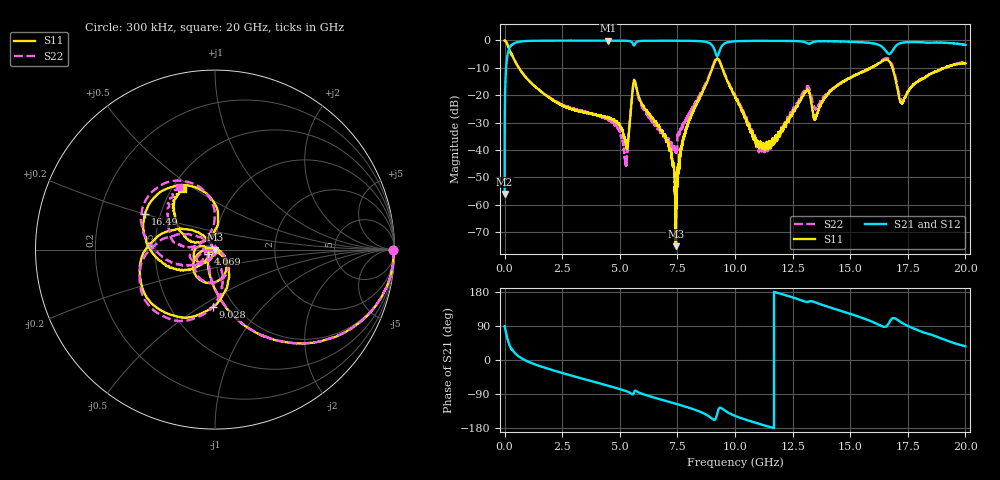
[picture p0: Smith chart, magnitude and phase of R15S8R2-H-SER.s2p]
!{R15S8R2}
!Johanson Technology Inc.
!www.johansontechnology.com
!Test Board Conditions:
!Substrate Type  RO4350B
!Substrate Thickness  20 mil
!Substrate Dk  3.66
!TL Type: GCPW
!TL Trace Width  34 mil
!TL Gap  10 mil
!Electrode orientation  Horizontal
!DUT TOPOLOGY	SERIES
!Mounting Pad LxW  26x52 mil
! Created Sat Feb  6 14:02:51 2021
# hz S ma R 50
! 2 Port Network Data from SP1.SP block
! freq  magS11  angS11  magS21  angS21  magS12  angS12  magS22  angS22
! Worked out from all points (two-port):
!   20001 points, 300 kHz to 20 GHz, reference 50 ohm
!   highest |S21| = -0.04 dB at 4.482 GHz (marker M1); lowest = -56.1 dB at 300 kHz (marker M2)
!   |S21| within 3 dB of the highest: 196.3 MHz to 9.091 GHz (8.895 GHz wide, 192 % of centre); 9.368 GHz to 16.47 GHz (7.102 GHz wide, 55 % of centre)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
!   lowest |S11| = -75.2 dB at 7.426 GHz (marker M3), VSWR 1.00, Z = 50 - j0.0107 ohm
!   |S11| at or under -10 dB: 618.2 MHz to 9.022 GHz (8.404 GHz wide, 174 % of centre); 9.44 GHz to 15.9 GHz (6.46 GHz wide, 51 % of centre); 16.83 GHz to 19.1 GHz (2.261 GHz wide, 12.6 % of centre)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
!   |S22| runs from -45.8 to 0.0 dB; largest |S21 - S12| = 0.017
!   S11 on the Smith chart (normalised r, x): 300 kHz: open; 4.069 GHz: 0.93, -0.04; 9.028 GHz: 0.80, -0.57; 16.49 GHz: 0.41, +0.20; 20 GHz: 0.57, +0.45
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300000  0.993 -0.1  0.00156 89.6  0.001487 90.3  0.9931 -0.1
1.093e8  0.87 -31.0  0.4865 58.8  0.4875 58.8  0.8712 -30.8
2.853e8  0.5627 -59.8  0.8177 29.6  0.8187 29.6  0.5627 -59.5
3.3343e9  0.04987 -139.7  0.9932 -48.5  0.9938 -48.5  0.05151 -139.5
4.0693e9  0.04297 -147.9  0.9941 -60.8  0.9935 -60.8  0.0424 -155.1
4.4823e9  0.03926 -152.4  0.9951 -67.7  0.993 -67.8  0.03648 -162.9
5.2623e9  0.01318 -130.1  0.9854 -81.9  0.9857 -81.9  0.005467 -117.6
5.6493e9  0.1857 -121.5  0.8417 -81.5  0.8422 -81.5  0.1808 -118.6
6.6673e9  0.02771 162.5  0.9879 -102.2  0.9869 -102.1  0.0243 -171.1
7.1523e9  0.009921 151.3  0.9877 -110.6  0.9877 -110.6  0.01275 -152.7
7.4263e9  0.0001736 -142.1  0.9868 -115.4  0.987 -115.4  0.009512 -119.9
7.8303e9  0.0201 -15.3  0.9849 -122.8  0.9859 -122.7  0.03274 -81.9
9.0283e9  0.3209 -92.0  0.7928 -156.0  0.7953 -156.0  0.3396 -95.2
9.3053e9  0.4303 -166.5  0.5969 -127.9  0.601 -128.1  0.445 -160.7
1.00003e10  0.09479 129.3  0.9655 -147.4  0.9661 -147.4  0.1002 138.7
1.12283e10  0.01278 -171.8  0.9823 -171.7  0.9809 -171.7  0.0117 21.4
1.30843e10  0.118 -149.0  0.9121 153.4  0.9119 153.4  0.1362 -147.0
1.33343e10  0.06355 163.2  0.913 155.3  0.9123 155.3  0.08592 171.5
1.64883e10  0.4384 152.9  0.6903 87.5  0.6842 88.1  0.4641 150.8
1.66673e10  0.4264 125.4  0.5685 96.0  0.5575 96.8  0.4639 127.3
1.72383e10  0.07184 128.0  0.905 98.6  0.9032 98.7  0.07917 131.0
2e10  0.3792 117.4  0.8354 36.1  0.8276 36.2  0.401 119.9
